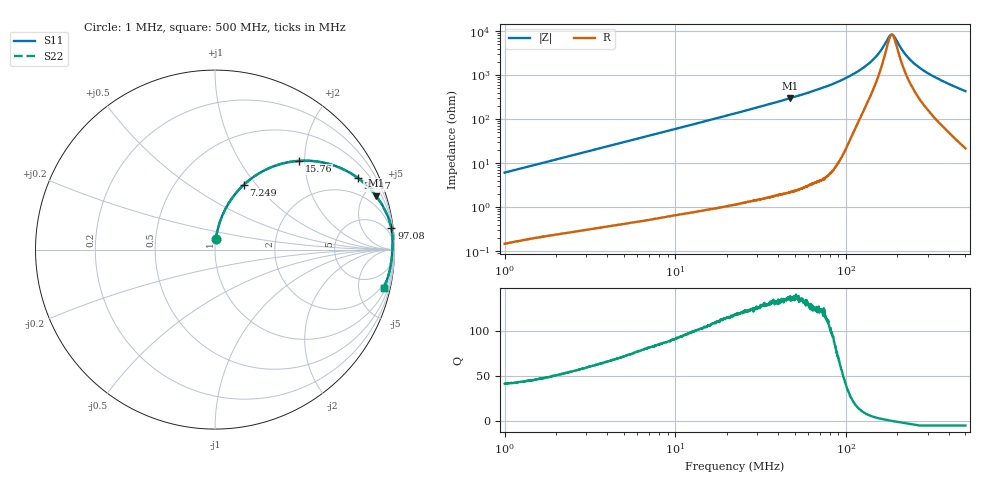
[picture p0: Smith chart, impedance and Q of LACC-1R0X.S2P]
!s-Parameter Generated by FASTRON Sdn. Bhd.
!FASTRON P/N : LACC-1R0X
!Keysight Technologies,E4991B,MY54100416,A.01.15
!Date: Mon Mar 30 13:18:02 2026
!Version  : Rev00 Mon Mar 30 13:18:02 2026
!Data & Calibration Information:
!PortZ  Port1:50+j0  Port2:50+j0
!When reading, reference impedance value at option line is always used.
!Remarks : This data is being provided solely for informational purposes.
!Freq	S11	S21	S12	S22
# Hz S dB R 50
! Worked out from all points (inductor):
!   1601 points, 1 MHz to 500 MHz, reference 50 ohm
!   read as one part in series: L = 965 nH near 1.032 MHz
!   highest Q = 138 at 46.95 MHz (marker M1), where L = 1.01 uH
!   self-resonance near 185.7 MHz
!   S11 on the Smith chart (normalised r, x): 1 MHz: 1.00, +0.12; 7.249 MHz: 1.01, +0.87; 15.76 MHz: 1.02, +1.88; 32.47 MHz: 1.03, +3.96; 97.08 MHz: 1, +16; 500 MHz: 1.43, -8.61
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1000000  -24.34 85.1  -0.03 -3.5  -0.03 -3.5  -24.34 85.1
2820919  -15.57 79.4  -0.15 -9.6  -0.15 -9.6  -15.57 79.4
4747111  -11.31 73.4  -0.37 -15.8  -0.37 -15.8  -11.31 73.4
7249310  -8.06 66.0  -0.78 -23.3  -0.78 -23.3  -8.06 66.0
7957584  -7.39 64.1  -0.92 -25.3  -0.92 -25.3  -7.39 64.1
1.576405e7  -3.32 46.4  -2.80 -43.0  -2.80 -43.0  -3.32 46.4
2.236068e7  -1.95 36.5  -4.52 -53.0  -4.52 -53.0  -1.95 36.5
3.246558e7  -1.01 26.7  -6.95 -62.9  -6.95 -62.9  -1.01 26.7
4.695421e7  -0.49 18.6  -9.94 -71.0  -9.94 -71.0  -0.49 18.6
6.307767e7  -0.25 13.3  -12.78 -76.3  -12.78 -76.3  -0.25 13.3
9.707707e7  -0.09 7.0  -18.28 -81.8  -18.28 -81.8  -0.09 7.0
1.197311e8  -0.08 4.4  -22.21 -81.2  -22.21 -81.2  -0.08 4.4
1.409467e8  -0.09 2.7  -26.40 -76.6  -26.40 -76.6  -0.09 2.7
1.577516e8  -0.09 1.6  -30.64 -67.8  -30.64 -67.8  -0.09 1.6
1.77937e8  -0.10 0.4  -37.34 -31.4  -37.34 -31.4  -0.10 0.4
1.842672e8  -0.10 0.1  -38.52 -6.3  -38.52 -6.3  -0.10 0.1
1.900828e8  -0.10 -0.2  -37.97 18.2  -37.97 18.2  -0.10 -0.2
2.263869e8  -0.12 -1.9  -28.83 67.4  -28.83 67.4  -0.12 -1.9
2.475421e8  -0.12 -2.9  -25.75 72.6  -25.75 72.6  -0.12 -2.9
2.770562e8  -0.14 -4.1  -22.81 75.6  -22.81 75.6  -0.14 -4.1
3.566264e8  -0.18 -7.2  -17.96 77.1  -17.96 77.1  -0.18 -7.2
5e8  -0.32 -12.9  -13.01 74.2  -13.01 74.2  -0.32 -12.9
